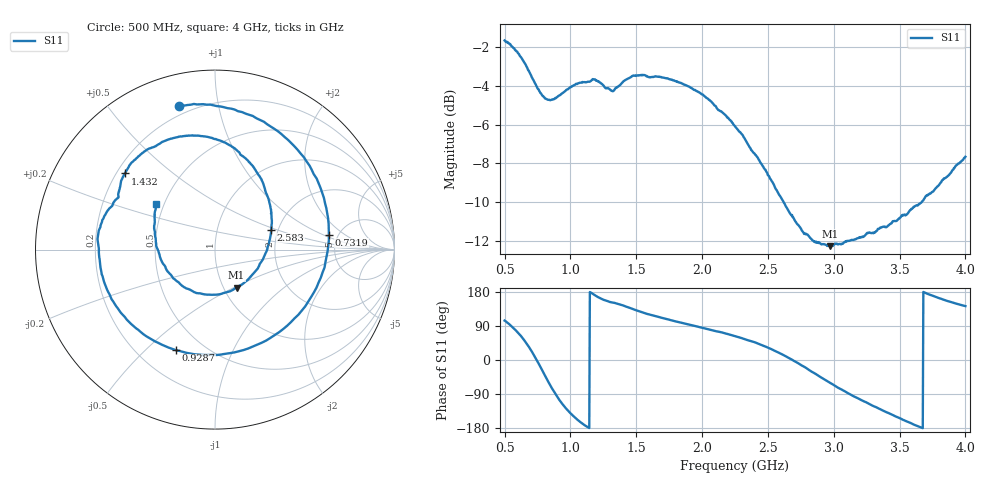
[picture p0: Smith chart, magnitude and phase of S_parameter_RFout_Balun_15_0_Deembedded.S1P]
!Agilent Technologies,E5071B,MY42403504,A.06.51
!Date: Wed Feb 26 14:58:16 2014
!Data & Calibration Information:
!Freq	S11:SOLT1(ON)
# Hz S dB R 50
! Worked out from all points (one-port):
!   801 points, 500 MHz to 4 GHz, reference 50 ohm
!   lowest |S11| = -12.3 dB at 2.972 GHz (marker M1), VSWR 1.64, Z = 57.5 - j25.8 ohm
!   |S11| at or under -10 dB: 2.619 GHz to 3.668 GHz (1.049 GHz wide, 33.4 % of centre)
!   S11 on the Smith chart (normalised r, x): 500 MHz: 0.15, +0.77; 731.9 MHz: 4.20, +1.19; 928.8 MHz: 0.35, -0.62; 1.432 GHz: 0.23, +0.35; 2.583 GHz: 1.84, +0.46; 4 GHz: 0.45, +0.28
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5e8  -1.65 104.0
5.65625e8  -2.04 85.0
6.225e8  -2.50 64.0
6.8375e8  -3.21 35.0
7.31875e8  -3.88 7.5
7.75625e8  -4.38 -20.5
8.325e8  -4.72 -58.0
8.7625e8  -4.68 -84.4
9.2875e8  -4.42 -111.4
9.375e8  -4.38 -115.4
1.011875e9  -4.02 -144.6
1.095e9  -3.81 -168.9
1.17375e9  -3.66 173.7
1.230625e9  -3.86 162.2
1.375e9  -3.97 146.6
1.431875e9  -3.64 139.8
1.571875e9  -3.46 122.8
1.8125e9  -3.79 100.8
2.009375e9  -4.47 84.4
2.25e9  -6.08 62.8
2.5825e9  -9.59 19.6
2.6875e9  -10.78 -0.2
2.971875e9  -12.28 -60.4
3.125e9  -11.99 -90.9
3.34375e9  -11.38 -128.3
3.5625e9  -10.58 -162.9
3.71125e9  -9.67 174.6
4e9  -7.66 142.3
